(* Logix 5000 AddOnInstructionDefinition export Banner_S15C_B21_PD_v4; software revision 33.00 *)

TYPE Banner_S15C_B21_PDI_v4 :   // UDT with all of the variables needed to control an IO-Link S15C-B21.
STRUCT
   Discrete_1_Status : SINT;   // 1 = Discrete 1 Active
   Discrete_2_Status : SINT;   // 1 = Discrete 2 Active
   Measurement_1 : DINT;
   Measurement_2 : DINT;
   Measurement_3 : DINT;
   Measurement_4 : DINT;
   DTI : SINT[18];   // Array with Raw Process data being transferred into AOI.
END_STRUCT
END_TYPE

ADD_ON_INSTRUCTION Banner_S15C_B21_PD_v4   (* revision 4.0, vendor Banner Engineering *)
// AOI that used with the S15C B21 sensor.
VAR_IN_OUT
   PD : Banner_S15C_B21_PDI_v4; {required}
END_VAR
VAR_INPUT
   Byte_Swap : BOOL; {required}
END_VAR
VAR
   Temp : SINT[18]; {access None}
END_VAR

ROUTINE Logic   (* ladder *)
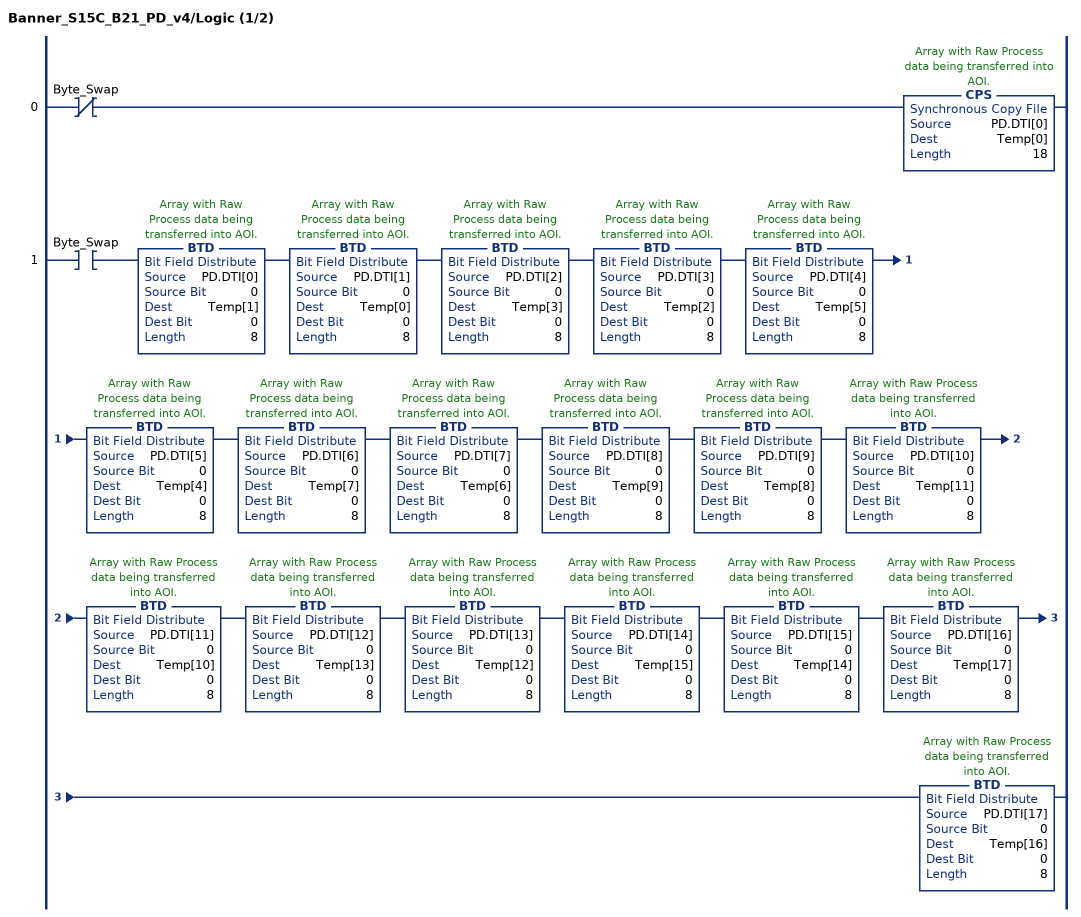
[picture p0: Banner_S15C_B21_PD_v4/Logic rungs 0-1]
   0: XIO(Byte_Swap)CPS(PD.DTI[0],Temp[0],18);
   1: XIC(Byte_Swap)BTD(PD.DTI[0],0,Temp[1],0,8)BTD(PD.DTI[1],0,Temp[0],0,8)BTD(PD.DTI[2],0,Temp[3],0,8)BTD(PD.DTI[3],0,Temp[2],0,8)BTD(PD.DTI[4],0,Temp[5],0,8)BTD(PD.DTI[5],0,Temp[4],0,8)BTD(PD.DTI[6],0,Temp[7],0,8)BTD(PD.DTI[7],0,Temp[6],0,8)BTD(PD.DTI[8],0,Temp[9],0,8)BTD(PD.DTI[9],0,Temp[8],0,8)BTD(PD.DTI[10],0,Temp[11],0,8)BTD(PD.DTI[11],0,Temp[10],0,8)BTD(PD.DTI[12],0,Temp[13],0,8)BTD(PD.DTI[13],0,Temp[12],0,8)BTD(PD.DTI[14],0,Temp[15],0,8)BTD(PD.DTI[15],0,Temp[14],0,8)BTD(PD.DTI[16],0,Temp[17],0,8)BTD(PD.DTI[17],0,Temp[16],0,8);
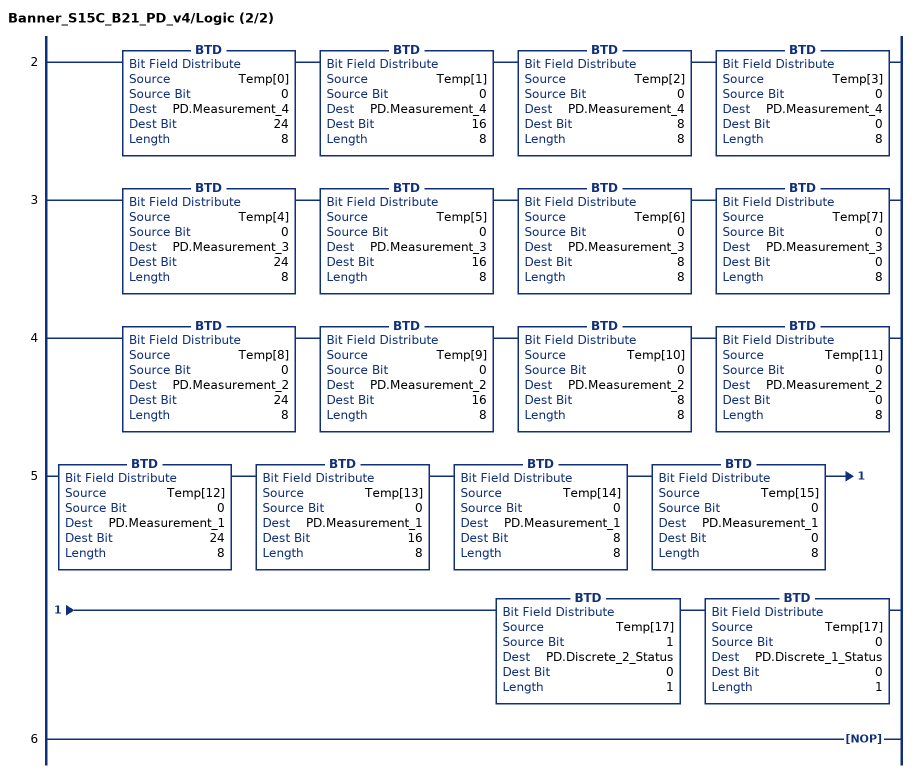
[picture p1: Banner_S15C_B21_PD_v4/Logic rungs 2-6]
   2: BTD(Temp[0],0,PD.Measurement_4,24,8)BTD(Temp[1],0,PD.Measurement_4,16,8)BTD(Temp[2],0,PD.Measurement_4,8,8)BTD(Temp[3],0,PD.Measurement_4,0,8);
   3: BTD(Temp[4],0,PD.Measurement_3,24,8)BTD(Temp[5],0,PD.Measurement_3,16,8)BTD(Temp[6],0,PD.Measurement_3,8,8)BTD(Temp[7],0,PD.Measurement_3,0,8);
   4: BTD(Temp[8],0,PD.Measurement_2,24,8)BTD(Temp[9],0,PD.Measurement_2,16,8)BTD(Temp[10],0,PD.Measurement_2,8,8)BTD(Temp[11],0,PD.Measurement_2,0,8);
   5: BTD(Temp[12],0,PD.Measurement_1,24,8)BTD(Temp[13],0,PD.Measurement_1,16,8)BTD(Temp[14],0,PD.Measurement_1,8,8)BTD(Temp[15],0,PD.Measurement_1,0,8)BTD(Temp[17],1,PD.Discrete_2_Status,0,1)BTD(Temp[17],0,PD.Discrete_1_Status,0,1);
   6: NOP();
END_ROUTINE
END_ADD_ON_INSTRUCTION
